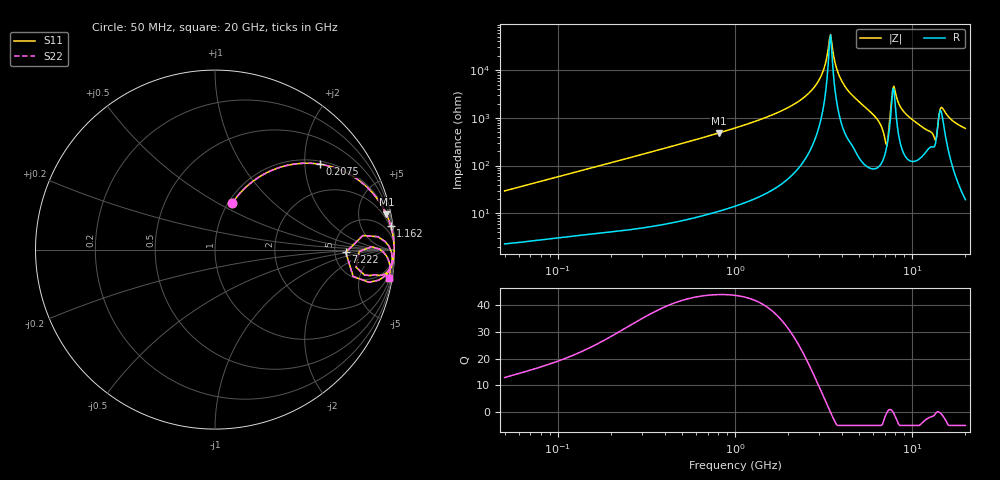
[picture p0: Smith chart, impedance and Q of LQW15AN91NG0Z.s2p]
!Murata Part Number: LQW15AN91NG0Z
!These Parameters are Measured in Series Mode Connection
!  o--[Z]--o
!Port1  Port2
!  o-------o
!Freq. Start=50[MHz] Stop=20[GHz], 401[Steps]
# Hz S RI R 50
!Freq.(Hz) S11(Real) S11(Imag) S21(Real) S21(Imag) S12(Real) S12(Imag) S22(Real) S22(Imag)
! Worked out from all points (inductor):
!   401 points, 50 MHz to 20 GHz, reference 50 ohm
!   read as one part in series: L = 93 nH near 51.52 MHz
!   highest Q = 43.9 at 810.8 MHz (marker M1), where L = 94.9 nH
!   self-resonance near 3.415 GHz
!   S11 on the Smith chart (normalised r, x): 50 MHz: 1.05, +0.59; 207.5 MHz: 1.08, +2.38; 1.162 GHz: 1, +15; 7.222 GHz: 6.35, -0.40; 20 GHz: 1, -12
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5e7  0.0966 0.2592  0.9034 -0.2592  0.9034 -0.2592  0.0966 0.2592
1.364002e8  0.3874 0.4656  0.6126 -0.4656  0.6126 -0.4656  0.3874 0.4656
2.074719e8  0.5839 0.4759  0.4161 -0.4759  0.4161 -0.4759  0.5839 0.4759
3.721004e8  0.8145 0.3758  0.1855 -0.3758  0.1855 -0.3758  0.8145 0.3758
8.108264e8  0.9548 0.1966  0.0452 -0.1966  0.0452 -0.1966  0.9548 0.1966
1e9  0.9706 0.1578  0.0294 -0.1578  0.0294 -0.1578  0.9706 0.1578
1.161586e9  0.9787 0.1331  0.0213 -0.1331  0.0213 -0.1331  0.9787 0.1331
1.99176e9  0.9944 0.0604  0.00561 -0.0604  0.00561 -0.0604  0.9944 0.0604
2.728004e9  0.9977 0.0255  0.00233 -0.0255  0.00233 -0.0255  0.9977 0.0255
3.121702e9  0.9982 0.011  0.0018 -0.011  0.0018 -0.011  0.9982 0.011
3.466789e9  0.9982 -0.000308  0.00175 0.000308  0.00175 0.000308  0.9982 -0.000308
3.792786e9  0.998 -0.0103  0.002 0.0103  0.002 0.0103  0.998 -0.0103
4.149438e9  0.9974 -0.0208  0.00265 0.0208  0.00265 0.0208  0.9974 -0.0208
6.217679e9  0.9831 -0.0938  0.0169 0.0938  0.0169 0.0938  0.9831 -0.0938
6.905011e9  0.9112 -0.1704  0.0888 0.1704  0.0888 0.1704  0.9112 -0.1704
7.222371e9  0.7287 -0.0148  0.2713 0.0148  0.2713 0.0148  0.7287 -0.0148
7.442007e9  0.9074 0.0719  0.0926 -0.0719  0.0926 -0.0719  0.9074 0.0719
7.901521e9  0.9817 -0.0109  0.0183 0.0109  0.0183 0.0109  0.9817 -0.0109
9.178299e9  0.9837 -0.0784  0.0163 0.0784  0.0163 0.0784  0.9837 -0.0784
1.314879e10  0.8663 -0.1446  0.1337 0.1446  0.1337 0.1446  0.8663 -0.1446
1.482269e10  0.9596 -0.0436  0.0404 0.0436  0.0404 0.0436  0.9596 -0.0436
2e10  0.9682 -0.16  0.0318 0.16  0.0318 0.16  0.9682 -0.16
